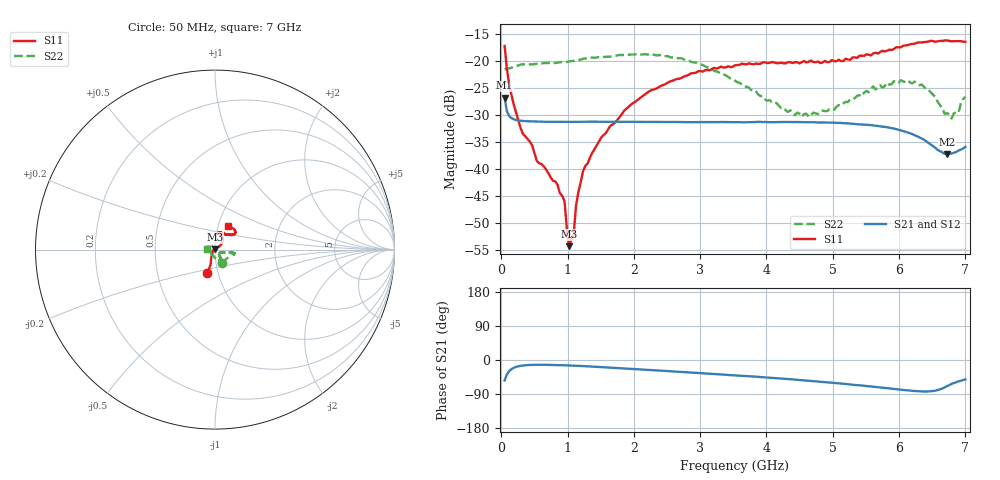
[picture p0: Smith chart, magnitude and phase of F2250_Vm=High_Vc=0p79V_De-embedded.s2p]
! Integrated Device Technology
! Corporate Headquarters
! 6024 Silver Creek Valley Road
! San Jose, CA 95138  USA
! Phone:  1-408-284-8200
! Toll Free:  1-800-223-1366
! Webpage:  http://www.idt.com/
! Timing and RF Division
! 515 Groton Road, Suite 102
! Westford, MA 01886-6024
! Device:  F2250
! Description: Voltage Variable RF Attenuator
! Frequency:  50.0 -  6000.00 MHz
! Package:  3x3 mm Thin QFN Plastic Package: 16 pin
! Ports:  2 RF, 3 DC
!  Pin  1  = GND
!  Pin  2  = NC
!  Pin  3  = RF1  = Port 1
!  Pin  4  = NC
!  Pin  5  = GND
!  Pin  6  = GND
!  Pin  7  = GND
!  Pin  8  = GND
!  Pin  9  = NC
!  Pin 10  = RF2  = Port 2
!  Pin 11  = NC
!  Pin 12  = GND
!  Pin 13  = GND
!  Pin 14  = VCNTRL
!  Pin 15  = VDD
!  Pin 16  = VMODE
! Vcntrl:  0.790 Volts
! Vmode:  +3.300 Volts
! Vdd:  +3.30  Volts
! Current:  1.299 mA
! Data:  The device was measured on a the F2250 evaluation board which has
!  individual transmission lines to the RF pins.  Data was collected
!  using a calibrated network analyzer.  The evaluation board was
!  de-embedded using a TRL calibration technique.
!  The reference plane is the edge of the package pin.
! Misc:  SN 10
!  Action Tracker AT0258
! Date Measured:  2014-11-26
! Date:  2015-10-15  MJV
! Note:
!  Integrated Device Technology supplies this data as a sample of measured
!  data at the package pin for this product.  Your particular data for this
!  product may vary.
!  Data was taken at 25 degrees C.
!  Integrated Device Technology reserves the right to change this data at anytime.
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# GHz S dB R 50
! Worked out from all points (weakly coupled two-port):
!   201 points, 50 MHz to 7 GHz, reference 50 ohm
!   highest |S21| = -26.75 dB at 50 MHz (marker M1); lowest = -37.2 dB at 6.722 GHz (marker M2)
!   lowest |S11| = -54.2 dB at 1.023 GHz (marker M3), VSWR 1.00, Z = 49.9 + j0.148 ohm
!   |S11| at or under -10 dB: start of sweep to end of sweep
!   |S22| runs from -30.6 to -18.7 dB; largest |S21 - S12| = 0.0001
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0.05  -17.14 -107.7  -26.75 -53.9  -26.76 -54.0  -21.50 -63.2
0.1195  -24.20 -110.9  -30.13 -29.3  -30.13 -29.3  -21.26 -19.6
0.29325  -32.42 -125.0  -31.00 -15.4  -31.00 -15.4  -20.58 -10.4
0.467  -35.62 -143.4  -31.12 -12.8  -31.12 -12.8  -20.57 -7.7
0.5365  -38.46 -151.4  -31.14 -12.6  -31.13 -12.6  -20.44 -8.4
0.8145  -42.22 171.0  -31.20 -13.2  -31.21 -13.2  -20.30 -10.6
0.9535  -45.85 173.1  -31.21 -14.0  -31.21 -14.0  -20.20 -11.9
1.023  -54.22 130.3  -31.21 -14.4  -31.22 -14.4  -20.01 -12.0
1.0925  -51.99 67.4  -31.21 -14.9  -31.22 -14.9  -19.93 -12.2
1.12725  -46.70 48.4  -31.20 -15.1  -31.21 -15.1  -19.80 -12.8
1.2315  -40.38 35.0  -31.19 -16.0  -31.17 -16.0  -19.53 -14.0
1.6485  -31.90 39.0  -31.18 -20.1  -31.19 -20.1  -19.13 -13.9
2.37825  -24.74 45.7  -31.23 -27.8  -31.23 -27.8  -18.83 -12.4
3.525  -20.71 71.2  -31.27 -40.5  -31.26 -40.6  -23.59 -13.6
4.4285  -20.17 74.3  -31.23 -51.7  -31.22 -51.8  -29.99 -34.1
4.7065  -20.14 71.7  -31.27 -55.7  -31.27 -55.8  -29.48 -43.0
5.85325  -17.83 40.2  -32.29 -75.0  -32.29 -75.1  -24.32 -58.6
6.33975  -16.50 40.5  -34.29 -82.8  -34.25 -83.0  -24.29 -72.6
6.722  -16.13 49.1  -37.16 -68.9  -37.17 -68.9  -29.58 -124.8
6.7915  -16.28 51.0  -37.07 -63.1  -37.07 -63.2  -30.58 -142.5
6.89575  -16.25 56.1  -36.49 -56.3  -36.47 -56.4  -29.50 -168.3
7  -16.38 62.1  -35.82 -51.1  -35.79 -51.3  -26.57 173.5
